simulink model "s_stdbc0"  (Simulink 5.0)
settings: Solver=ode45  SolverMode=SingleTasking  StartTime=0.0  StopTime=200.0  MaxStep=0.4  RelTol=1e-3  AbsTol=1e-6

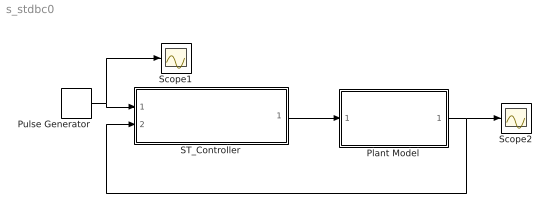
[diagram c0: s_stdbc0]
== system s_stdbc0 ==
  Plant Model : Subsystem
  Pulse Generator : DiscretePulseGenerator  PulseType=Time based  Period=300  PulseWidth=50
  ST_Controller : Subsystem  mask(ST_Controller){B=[0 0 2], A=[5 3 6], ff=0.9, pdiag=10000, ts=10}
      mask prompts: B "Numerator :"; A "Denominator  :"; ff "Forgetting factor ff :"; pdiag "Covariance matrix diagonal elements :"; ts "How often to sample points [sec] ;"
      mask help: Adaptiven aperiodichen regulator, imasht poriadaka na sistemata, koiato se regulira i zadava s chislitel B i znamenatel A:
      mask init:
      | B=@1; A=@2; ff=@3; pdiag=@4; ts=@5; format short g;
      | Q=B; P=A;  order=2;  na=2; nb=2; nk=1;  nn=[na nb nk];
      |   format short g;
  Scope1 : Scope
  Scope2 : Scope
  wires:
  Plant Model/1(Out1) -> ST_Controller/2(In2), Scope2/1
  ST_Controller/1(Out2) -> Plant Model/1(In1)
  Pulse Generator/1 -> ST_Controller/1(In1), Scope1/1

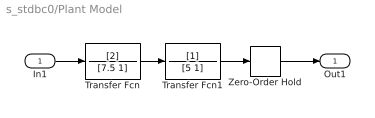
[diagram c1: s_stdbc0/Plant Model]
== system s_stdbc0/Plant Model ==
  In1 : Inport
  Transfer Fcn : TransferFcn  Numerator=[2]  Denominator=[7.5 1]
  Transfer Fcn1 : TransferFcn  Denominator=[5 1]
  Zero-Order Hold : ZeroOrderHold
  Out1 : Outport  InitialOutput=0
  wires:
  Transfer Fcn/1 -> Transfer Fcn1/1
  Transfer Fcn1/1 -> Zero-Order Hold/1
  Zero-Order Hold/1 -> Out1/1
  In1/1 -> Transfer Fcn/1

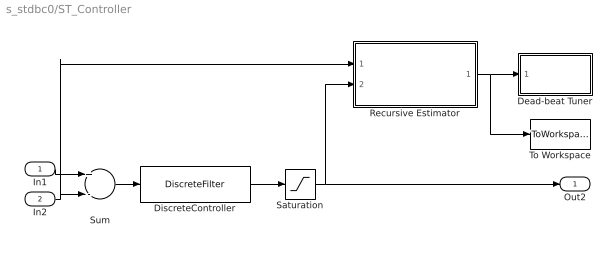
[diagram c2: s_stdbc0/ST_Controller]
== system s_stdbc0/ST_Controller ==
  In1 : Inport
  In2 : Inport  Port=2
  Dead-beat Tuner : Subsystem  mask(DBC Tuner){name=['s_stdbc0/ST_Controller/DiscreteController'], order=order}
      mask prompts: name "Regulator name ['string' ]:"; order "Namber parameters :"
      mask help: Blok za nastrojka na diskreten regulator. Izpolzva S-function ab2pq_sl.
      mask init:
      | name=@1; order=@2;
  DiscreteController : DiscreteFilter  Numerator=[0 2.22044605101768e-016 2.22044605102869e-016]  Denominator=[1 -2.22044604572913e-016 -2.22044604577783e-016]
  Recursive Estimator : Subsystem  mask(Recursive Estimator){nn=[na nb nk], ff=ff, pdiag=pdiag, ts=ts}
      mask prompts: nn "ARX model structure [na nb nk]  :"; ff "Forgetting factor  ff :"; pdiag "Initial value for the diagonal of covariance matrix P :"; ts "How often to sample points [sec] :"
      mask help: Recursive parameter estimation
      mask init:
      | nn=@1; ff=@2; pdiag=@3; ts=@4;
      | na=nn(1); nb=nn(2); nk=nn(3); d=na+nb; dm=sum(nn)-1;
      | i=[1:na  na+nk:dm];  ii=[1:dm];
  Saturation : Saturate  UpperLimit=125  LowerLimit=-125
  Sum : Sum  Inputs=+-
  To Workspace : ToWorkspace  VariableName=th_est  SampleTime=-1  SaveFormat=Array
  Out2 : Outport
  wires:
  Sum/1 -> DiscreteController/1
  In1/1 -> Sum/1
  In2/1 -> Sum/2, Recursive Estimator/1(y (k))
  Recursive Estimator/1(tetha (k)) -> To Workspace/1, Dead-beat Tuner/1(In1)
  DiscreteController/1 -> Saturation/1
  Saturation/1 -> Out2/1, Recursive Estimator/2(u (k))

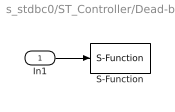
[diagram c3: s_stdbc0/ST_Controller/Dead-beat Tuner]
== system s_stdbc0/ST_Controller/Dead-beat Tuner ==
  In1 : Inport
  S-Function : S-Function  FunctionName=ab2pq_sl  Parameters=name,order
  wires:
  In1/1 -> S-Function/1

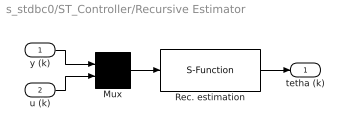
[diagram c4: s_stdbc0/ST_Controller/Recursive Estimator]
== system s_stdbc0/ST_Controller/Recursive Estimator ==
  y (k) : Inport
  u (k) : Inport  Port=2
  Mux : Mux  Inputs=2
  Rec. estimation : S-Function  FunctionName=rarxm_sl  Parameters=na, ff,pdiag,ts,d,dm,i,ii
  tetha (k) : Outport
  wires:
  Rec. estimation/1 -> tetha (k)/1
  Mux/1 -> Rec. estimation/1
  u (k)/1 -> Mux/2
  y (k)/1 -> Mux/1
